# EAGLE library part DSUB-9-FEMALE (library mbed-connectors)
DSUB-Connector female 9-pol
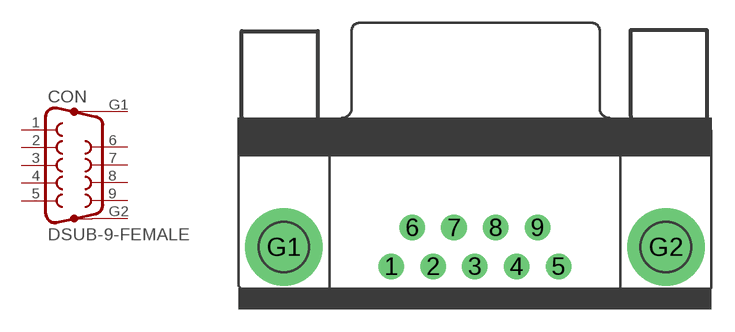
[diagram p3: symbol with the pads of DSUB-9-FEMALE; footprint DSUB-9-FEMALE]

Designator prefix CON

## DSUB-9-FEMALE  [DSUB-9-FEMALE]
1  1  pas
2  2  pas
3  3  pas
4  4  pas
5  5  pas
6  6  pas
7  7  pas
8  8  pas
9  9  pas
G1  G1  pas
G2  G2  pas

## Footprint DSUB-9-FEMALE (pad centres in mm)
DSUB Connector female 9-pol
drill 1.016 pad 1.676: 1 -5.486,-1.524; 2 -2.743,-1.524; 3 0,-1.524; 4 2.743,-1.524; 5 5.486,-1.524; 6 -4.115,1.016; 7 -1.372,1.016; 8 1.372,1.016; 9 4.115,1.016
drill 3.302 pad 5.08: G1 -12.522,-0.254; G2 12.522,-0.254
